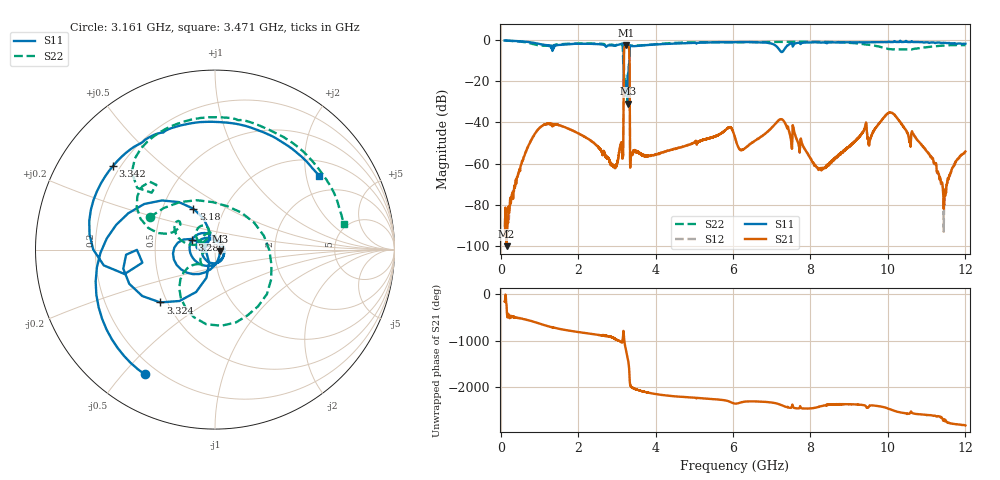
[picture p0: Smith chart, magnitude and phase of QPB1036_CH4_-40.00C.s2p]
! TDS: K:\Engsetup\Winsaw\QPB1036_ALL
! Channel 1
! Ports=1 2
! seg 1=100.000000 1100.000000 101
! seg 2=1101.000000 1501.000000 401
! seg 3=1502.000000 2502.000000 101
! seg 4=2503.000000 3803.000000 1301
! seg 5=3804.000000 5004.000000 121
! seg 6=5005.000000 6005.000000 1001
! seg 7=6006.000000 8406.000000 241
! seg 8=8407.000000 10607.000000 2201
! seg 9=10608.000000 12008.000000 141
! Points=5609
! FailCode=0
! Topology=ALL_SE(12)
!VNA Cal loaded =QPB1036_ALL_-40C
!PS1(V)= 5.000
!PS(mA)= 0.500
!PS2(V)= 1.170
!PS(mA)= -0.100
!PS3(V)= 0.630
!PS(mA)= 0.100
!PS4(V)= 0.630
!PS(mA)= -0.100
!Temp (C)= -40.00
# MHz S DB R 50
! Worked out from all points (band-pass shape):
!   5609 points, 100 MHz to 12.01 GHz, reference 50 ohm
!   highest |S21| = -2.42 dB at 3.24 GHz (marker M1); lowest = -100.0 dB at 150 MHz (marker M2)
!   |S21| within 3 dB of the highest: 3.187 GHz to 3.321 GHz (134.7 MHz wide, 4.14 % of centre)
!   lowest |S11| = -30.8 dB at 3.301 GHz (marker M3), VSWR 1.06, Z = 52.8 - j0.93 ohm
!   |S11| at or under -10 dB: 3.179 GHz to 3.323 GHz (143.5 MHz wide, 4.41 % of centre)
!   |S22| runs from -29.5 to -0.3 dB; largest |S21 - S12| = 0.0071
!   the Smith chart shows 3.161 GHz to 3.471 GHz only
!   S11 on the Smith chart (normalised r, x): 3.161 GHz: 0.15, -0.57; 3.18 GHz: 0.71, +0.35; 3.289 GHz: 0.77, +0.09; 3.324 GHz: 0.46, -0.33; 3.342 GHz: 0.17, +0.35; 3.471 GHz: 1.43, +2.38
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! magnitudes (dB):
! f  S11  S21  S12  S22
! 100 MHz  -0.2  -94.9  -90.6  -0.3
! 150 MHz  -0.3  -100.0  -94.1  -0.3
! 1.125 GHz  -2.4  -41.1  -41.1  -2.8
! 2.092 GHz  -1.8  -46.1  -46.1  -1.7
! 2.959 GHz  -2.8  -61.8  -61.7  -2.8
! 3.139 GHz  -1.7  -55.5  -55.3  -2.3
! 3.161 GHz  -2.0  -55.6  -55.7  -7.8
! 3.18 GHz  -11.8  -10.8  -10.8  -8.8
! 3.24 GHz  -22.9  -2.4  -2.4  -21.5
! 3.289 GHz  -17.1  -2.9  -2.9  -16.3
! 3.301 GHz  -30.8  -3.2  -3.1  -22.0
! 3.324 GHz  -7.5  -7.1  -7.1  -7.0
! 3.342 GHz  -2.7  -57.7  -57.7  -2.7
! 3.367 GHz  -2.9  -56.4  -56.1  -2.7
! 3.471 GHz  -3.0  -53.6  -54.0  -2.7
! 4.074 GHz  -2.1  -55.1  -55.1  -2.0
! 6.056 GHz  -1.1  -47.4  -47.5  -1.1
! 7.206 GHz  -4.9  -38.6  -38.6  -0.9
! 8.046 GHz  -1.1  -58.8  -58.7  -0.9
! 10.02 GHz  -0.8  -35.3  -35.4  -4.4
! 11.39 GHz  -1.4  -69.5  -68.8  -2.8
! 12.01 GHz  -1.9  -54.1  -54.5  -2.5
